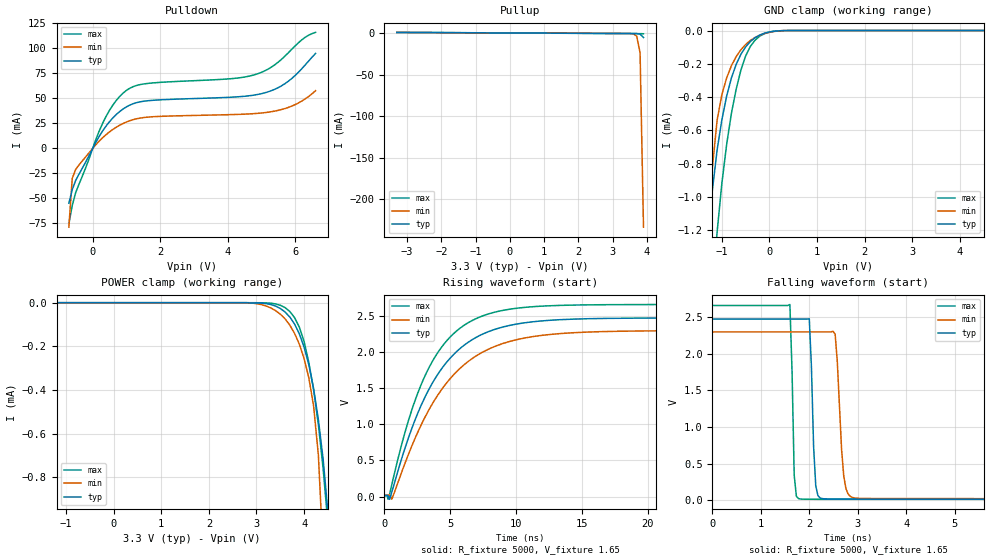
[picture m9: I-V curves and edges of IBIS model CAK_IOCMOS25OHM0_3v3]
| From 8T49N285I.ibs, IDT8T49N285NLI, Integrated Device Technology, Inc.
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[Model] CAK_IOCMOS25OHM0_3v3
Model_type   I/O
Polarity   Non-Inverting
|   typ   min   max
C_comp   2pF   1.5pF   2.5pF
|Input
Vinl = 0.8V
Vinh = 2.0V
|Output
Vmeas = 1.65V
Rref = 5000
Cref = 0
Vref = 1.65V
|   typ   min   max
[Voltage range]   3.3V   3.135V   3.465V
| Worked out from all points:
|   slope of the pulldown table from 0 to 0.495 V, typ, clamps not added: 18.6 ohm
|   slope of the pullup table from 0 to 0.495 V, typ, clamps not added: 5.02 kohm
|   GND clamp passes 1 mA (typ) near -1.21 V on its own axis
|   rising waveform, R_fixture 5000, V_fixture 1.65: 20-80 % time 4.06ns typ, 4.58ns min, 3.55ns max; typ from 0.014 V to 2.47 V
|   falling waveform, R_fixture 5000, V_fixture 1.65: 20-80 % time 74.4ps typ, 111ps min, 56.2ps max; typ from 2.47 V to 0.014 V
[GND_clamp]
|Voltage   I (typ)   I (min)   I (max)
|Note, modeling breaks down at 250mA and above.  This is well beyond the functional   |
|operating range of the device.  Should this scenario occur, catastrophic failure and   |
|possible damage to the device and/or board is of higher concern than the I-V curve   |
|behavior.  The IBIS checker will flag currents in excess of 10A with warnings.  Lines   |
|with currents in excess of 0.35 A have been commented out.  The points still remain|
|available to the user if the user desires to use them.   |
|-3.30000e+00   -1.93906e+00   -1.61999e+00   -2.35041e+00
|-3.20000e+00   -1.77927e+00   -1.50039e+00   -2.14297e+00
|-3.10000e+00   -1.62023e+00   -1.38139e+00   -1.93638e+00
|-3.00000e+00   -1.46206e+00   -1.26306e+00   -1.73086e+00
|-2.90000e+00   -1.30490e+00   -1.14549e+00   -1.52658e+00
|-2.80000e+00   -1.14902e+00   -1.02915e+00   -1.32384e+00
|-2.70000e+00   -9.94687e-01   -9.12920e-01   -1.12308e+00
|-2.60000e+00   -8.41736e-01   -7.98445e-01   -9.25435e-01
|-2.50000e+00   -6.91717e-01   -6.85656e-01   -7.30530e-01
|-2.40000e+00   -5.45423e-01   -5.75028e-01   -5.41495e-01
|-2.30000e+00   -4.04669e-01   -4.67289e-01   -3.62221e-01
|-2.20000e+00   -2.72864e-01   -3.63595e-01   -2.00956e-01
-2.1V     -156.9mA   -265.8mA   -87.23mA
-1.3V     -1.329mA   -1.412mA   -2.197mA
-1.2V     -961uA     -826.1uA   -1.616mA
-1.1V     -717.9uA   -539.1uA   -1.212mA
-1V       -536.6uA   -385.3uA   -918.2uA
-900mV    -394.5uA   -285.1uA   -685.5uA
-800mV    -285.3uA   -211.7uA   -498.5uA
-700mV    -203.6uA   -157uA     -353.2uA
-500mV    -98.11uA   -83.66uA   -152.3uA
-200mV    -26.47uA   -27.83uA   -33.08uA
300mV     -639.8nA   -237nA     -586.4nA
6.6V      10.83nA    21.6nA     10.26nA
[Power_clamp]
|Voltage   I (typ)   I (min)   I (max)
|Note, modeling breaks down at 250mA and above.  This is well beyond the functional   |
|operating range of the device.  Should this scenario occur, catastrophic failure and   |
|possible damage to the device and/or board is of higher concern than the I-V curve   |
|behavior.  The IBIS checker will flag currents in excess of 10A with warnings.  Lines   |
|with currents in excess of 0.35 A have been commented out.  The points still remain|
|available to the user if the user desires to use them.   |
-3.3V     9.4nA      17.43nA    13.8nA
2.8V      -30.97nA   -86.03nA   -40.38pA
3.2V      -4.061uA   -14.87uA   -854.1nA
3.5V      -26.47uA   -52.46uA   -11.68uA
3.7V      -65.72uA   -103uA     -40.28uA
3.9V      -142.6uA   -190.2uA   -112.2uA
4.1V      -285.3uA   -345.3uA   -274.4uA
4.2V      -394.5uA   -474uA     -400.2uA
4.3V      -536.6uA   -699.3uA   -559uA
4.4V      -717.9uA   -1.15mA    -761.4uA
4.5V      -961uA     -2.088mA   -1.012mA
5.3V      -71.96mA   -327.6mA   -24.7mA
| 5.40000e+00   -1.56891e-01   -4.29414e-01   -3.52385e-02
| 5.50000e+00   -2.72864e-01   -5.35861e-01   -5.17705e-02
| 5.60000e+00   -4.04669e-01   -6.45549e-01   -1.16666e-01
| 5.70000e+00   -5.45423e-01   -7.57626e-01   -2.54470e-01
| 5.80000e+00   -6.91717e-01   -8.71535e-01   -4.23484e-01
| 5.90000e+00   -8.41736e-01   -9.86981e-01   -6.06782e-01
| 6.00000e+00   -9.94687e-01   -1.10343e+00   -7.98616e-01
| 6.10000e+00   -1.14902e+00   -1.22064e+00   -9.94106e-01
| 6.20000e+00   -1.30490e+00   -1.33871e+00   -1.19308e+00
| 6.30000e+00   -1.46206e+00   -1.45748e+00   -1.39461e+00
| 6.40000e+00   -1.62023e+00   -1.57687e+00   -1.59792e+00
| 6.50000e+00   -1.77927e+00   -1.69679e+00   -1.80266e+00
| 6.60000e+00   -1.93906e+00   -1.81717e+00   -2.00858e+00
[Pulldown]
|Voltage   I (typ)   I (min)   I (max)
|Note, modeling breaks down at 250mA and above.  This is well beyond the functional   |
|operating range of the device.  Should this scenario occur, catastrophic failure and   |
|possible damage to the device and/or board is of higher concern than the I-V curve   |
|behavior.  The IBIS checker will flag currents in excess of 10A with warnings.  Lines   |
|with currents in excess of 0.35 A have been commented out.  The points still remain|
|available to the user if the user desires to use them.   |
|-3.300000e+00   -1.633864e+01   -1.284091e+01   -2.022129e+01
|-3.200000e+00   -1.574873e+01   -1.239821e+01   -1.947163e+01
|-3.100000e+00   -1.515817e+01   -1.195511e+01   -1.872102e+01
|-3.000000e+00   -1.456664e+01   -1.151124e+01   -1.796934e+01
|-2.900000e+00   -1.397420e+01   -1.106681e+01   -1.721642e+01
|-2.800000e+00   -1.338038e+01   -1.062115e+01   -1.646196e+01
|-2.700000e+00   -1.278511e+01   -1.017548e+01   -1.570542e+01
|-2.600000e+00   -1.218846e+01   -9.728155e+00   -1.494576e+01
|-2.500000e+00   -1.158888e+01   -9.279234e+00   -1.418337e+01
|-2.400000e+00   -1.098568e+01   -8.828212e+00   -1.341511e+01
|-2.300000e+00   -1.037683e+01   -8.374401e+00   -1.263698e+01
|-2.200000e+00   -9.759236e+00   -7.916635e+00   -1.184094e+01
|-2.100000e+00   -9.125729e+00   -7.453056e+00   -1.099727e+01
|-2.000000e+00   -8.461274e+00   -6.980146e+00   -1.008359e+01
|-1.900000e+00   -7.751551e+00   -6.495277e+00   -9.138122e+00
|-1.800000e+00   -7.016586e+00   -5.985001e+00   -8.191320e+00
|-1.700000e+00   -6.274624e+00   -5.450977e+00   -7.242611e+00
|-1.600000e+00   -5.530210e+00   -4.902866e+00   -6.290711e+00
|-1.500000e+00   -4.783930e+00   -4.347968e+00   -5.336026e+00
|-1.400000e+00   -4.036411e+00   -3.790123e+00   -4.379860e+00
|-1.300000e+00   -3.288341e+00   -3.231058e+00   -3.423283e+00
|-1.200000e+00   -2.540169e+00   -2.671524e+00   -2.466544e+00
|-1.100000e+00   -1.792092e+00   -2.111881e+00   -1.509758e+00
|-1.000000e+00   -1.044193e+00   -1.552335e+00   -5.530228e-01
|-9.000000e-01   -3.153515e-01   -9.930789e-01   -1.202065e-01
|-8.000000e-01   -7.666415e-02   -4.342823e-01   -9.606150e-02
-700mV    -54.94mA   -78.86mA   -75.69mA
-600mV    -41.52mA   -30.23mA   -57.3mA
-500mV    -32.38mA   -21.39mA   -44.53mA
300mV     17.14mA    10.35mA    24.78mA
600mV     30.03mA    18.55mA    42.8mA
1V        41.06mA    25.95mA    57.46mA
1.5V      46.66mA    30.39mA    63.87mA
4.2V      50.92mA    33.49mA    69.53mA
5.1V      55.15mA    35.37mA    77.11mA
5.8V      66.82mA    40.65mA    95.25mA
6.2V      79.44mA    47.06mA    108.2mA
6.6V      94.44mA    57.23mA    115.4mA
[Pullup]
|Voltage   I (typ)   I (min)   I (max)
|Note, modeling breaks down at 250mA and above.  This is well beyond the functional   |
|operating range of the device.  Should this scenario occur, catastrophic failure and   |
|possible damage to the device and/or board is of higher concern than the I-V curve   |
|behavior.  The IBIS checker will flag currents in excess of 10A with warnings.  Lines   |
|with currents in excess of 0.35 A have been commented out.  The points still remain|
|available to the user if the user desires to use them.   |
-3.3V     657.4uA    576uA      759.5uA
3.5V      -670.7uA   -596.9uA   -793.8uA
3.6V      -676.1uA   -974.5uA   -806uA
3.7V      -721.7uA   -3.732mA   -811.2uA
3.8V      -1.428mA   -23.61mA   -812.1uA
3.9V      -5.448mA   -233.6mA   -958.2uA
|4.000000e+00   -1.455248e-02   -7.663110e-01   -3.221085e-03
|4.100000e+00   -3.265685e-02   -1.323195e+00   -1.213237e-02
|4.200000e+00   -2.682705e-01   -1.880666e+00   -2.705835e-02
|4.300000e+00   -9.944094e-01   -2.438471e+00   -4.264551e-02
|4.400000e+00   -1.739912e+00   -2.996400e+00   -9.285493e-02
|4.500000e+00   -2.485879e+00   -3.554152e+00   -8.215286e-01
|4.600000e+00   -3.232201e+00   -4.111162e+00   -1.775704e+00
|4.700000e+00   -3.978651e+00   -4.666145e+00   -2.730283e+00
|4.800000e+00   -4.724790e+00   -5.216168e+00   -3.685122e+00
|4.900000e+00   -5.469880e+00   -5.755262e+00   -4.640089e+00
|5.000000e+00   -6.213294e+00   -6.274209e+00   -5.594663e+00
|5.100000e+00   -6.954406e+00   -6.766093e+00   -6.547506e+00
|5.200000e+00   -7.688691e+00   -7.241858e+00   -7.497484e+00
|5.300000e+00   -8.397834e+00   -7.707553e+00   -8.444646e+00
|5.400000e+00   -9.061829e+00   -8.166526e+00   -9.391021e+00
|5.500000e+00   -9.694916e+00   -8.621039e+00   -1.033153e+01
|5.600000e+00   -1.031233e+01   -9.072461e+00   -1.122373e+01
|5.700000e+00   -1.092078e+01   -9.521674e+00   -1.204313e+01
|5.800000e+00   -1.152388e+01   -9.969065e+00   -1.283142e+01
|5.900000e+00   -1.212326e+01   -1.041512e+01   -1.360542e+01
|6.000000e+00   -1.271981e+01   -1.086027e+01   -1.437088e+01
|6.100000e+00   -1.331498e+01   -1.130476e+01   -1.513269e+01
|6.200000e+00   -1.390870e+01   -1.174849e+01   -1.589102e+01
|6.300000e+00   -1.450114e+01   -1.219162e+01   -1.664679e+01
|6.400000e+00   -1.509257e+01   -1.263423e+01   -1.740078e+01
|6.500000e+00   -1.568323e+01   -1.307631e+01   -1.815334e+01
|6.600000e+00   -1.627304e+01   -1.351803e+01   -1.890462e+01
[Ramp]
|   typ   min   max
dV/dt_r   1.507/4.074n   1.4/4.593n   1.616/3.561n
dV/dt_f   1.477/0.074n   1.371/0.111n   1.596/0.056n
R_load =   50.0000
[Rising Waveform]
R_fixture = 5000
V_fixture = 1.65   |Vcc_typ
V_fixture_min = 1.5675 |Vcc_min
V_fixture_max = 1.7325 |Vcc_max
C_fixture = 0.0p
| Time   typ   min   max
0s        14.41mV    20.9mV     11.46mV
311.1ps   -1.519mV   20.99mV    -32mV
577.8ps   75.63mV    -31.06mV   181mV
2.044ns   925.9mV    684.5mV    1.18V
3.556ns   1.544V     1.258V     1.843V
5.289ns   1.973V     1.693V     2.262V
7.511ns   2.254V     2.005V     2.505V
10.4ns    2.399V     2.186V     2.615V
14.62ns   2.458V     2.271V     2.652V
40ns      2.473V     2.298V     2.659V
[Falling Waveform]
R_fixture = 5000
V_fixture = 1.65   |Vcc_typ
V_fixture_min = 1.5675 |Vcc_min
V_fixture_max = 1.7325 |Vcc_max
C_fixture = 0.0p
| Time   typ   min   max
0s        2.473V     2.298V     2.659V
1.6ns     2.473V     2.298V     2.673V
1.689ns   2.473V     2.298V     339.9mV
1.822ns   2.473V     2.298V     15.4mV
2ns       2.477V     2.298V     12.38mV
2.133ns   197.7mV    2.298V     12.04mV
2.311ns   18.31mV    2.298V     11.84mV
2.533ns   15.54mV    2.267V     11.71mV
2.978ns   14.86mV    26.86mV    11.59mV
40ns      14.41mV    20.9mV     11.46mV
